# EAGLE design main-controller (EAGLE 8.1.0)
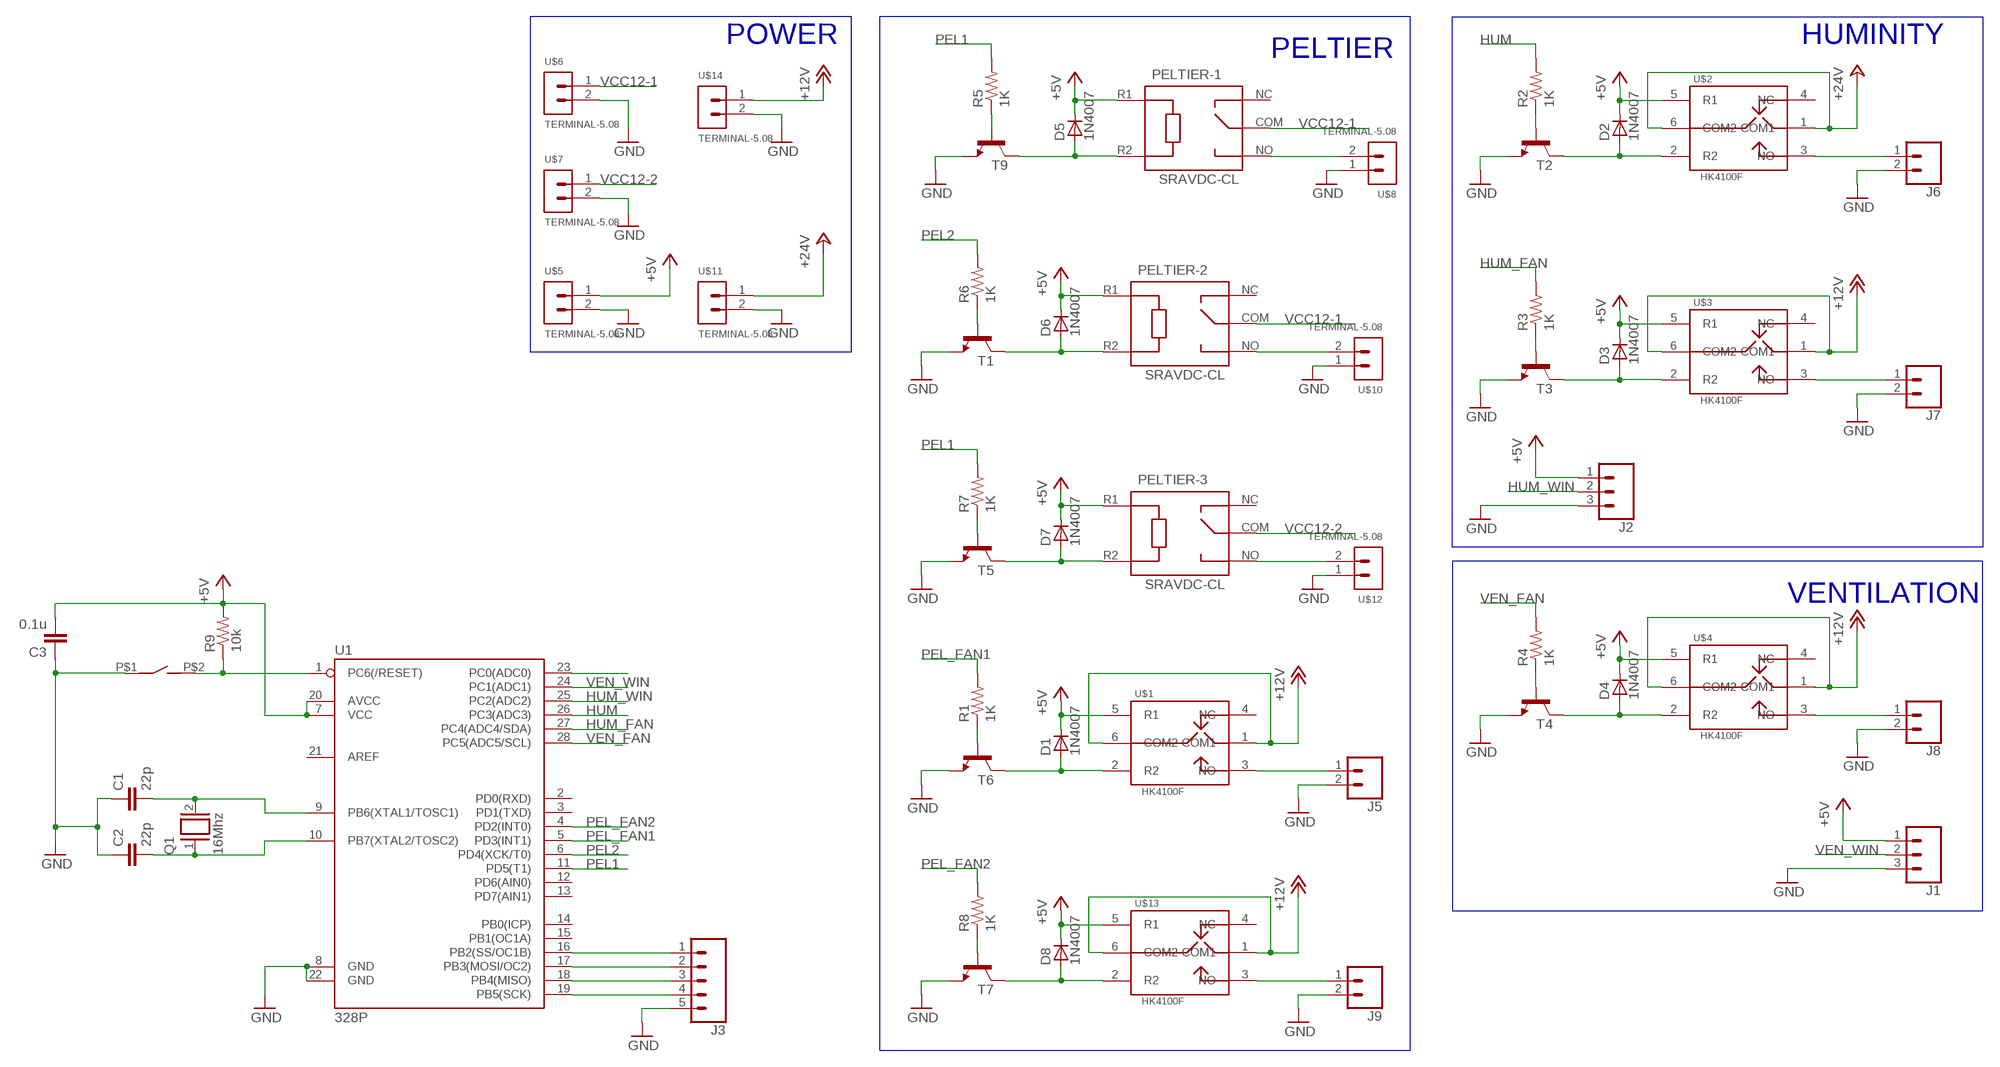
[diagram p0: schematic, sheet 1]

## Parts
C1  22p  C-EUC0805  [C0805]
C2  22p  C-EUC0805  [C0805]
C3  0.1u  C-EUC0805  [C0805]
D1  1N4007  [SMA]
D2  1N4007  [SMA]
D3  1N4007  [SMA]
D4  1N4007  [SMA]
D5  1N4007  [SMA]
D6  1N4007  [SMA]
D7  1N4007  [SMA]
D8  1N4007  [SMA]
J1  CONN_03  [1X03]
J2  CONN_03  [1X03]
J3  CONN_05KH2510  [1X05KF2510]
J5  CONN_02POLAR  [MOLEX-1X2]
J6  CONN_02POLAR  [MOLEX-1X2]
J7  CONN_02POLAR  [MOLEX-1X2]
J8  CONN_02POLAR  [MOLEX-1X2]
J9  CONN_02POLAR  [MOLEX-1X2]
PELTIER-1  SRAVDC-CL  [SRA-*VDC-CL]
PELTIER-2  SRAVDC-CL  [SRA-*VDC-CL]
PELTIER-3  SRAVDC-CL  [SRA-*VDC-CL]
Q1  16Mhz  XTAL/S  [QS]
R1  1K  R-US_M0805  [M0805]
R2  1K  R-US_M0805  [M0805]
R3  1K  R-US_M0805  [M0805]
R4  1K  R-US_M0805  [M0805]
R5  1K  R-US_M0805  [M0805]
R6  1K  R-US_M0805  [M0805]
R7  1K  R-US_M0805  [M0805]
R8  1K  R-US_M0805  [M0805]
R9  10k  R-US_R0805  [R0805]
T1  -NPN-SOT23-EBC  [SOT23-EBC]
T2  -NPN-SOT23-EBC  [SOT23-EBC]
T3  -NPN-SOT23-EBC  [SOT23-EBC]
T4  -NPN-SOT23-EBC  [SOT23-EBC]
T5  -NPN-SOT23-EBC  [SOT23-EBC]
T6  -NPN-SOT23-EBC  [SOT23-EBC]
T7  -NPN-SOT23-EBC  [SOT23-EBC]
T9  -NPN-SOT23-EBC  [SOT23-EBC]
U1  328P  ATMEGA328P_PDIP  [DIP28]
U$1  HK4100F  [HK4100F-DC5V-SHG]
U$2  HK4100F  [HK4100F-DC5V-SHG]
U$3  HK4100F  [HK4100F-DC5V-SHG]
U$4  HK4100F  [HK4100F-DC5V-SHG]
U$5  TERMINAL-5.08  [TERMINAL-5.08]
U$6  TERMINAL-5.08  [TERMINAL-5.08]
U$7  TERMINAL-5.08  [TERMINAL-5.08]
U$8  TERMINAL-5.08  [TERMINAL-5.08]
U$9  BUTTON  [BUTTON-2]
U$10  TERMINAL-5.08  [TERMINAL-5.08]
U$11  TERMINAL-5.08  [TERMINAL-5.08]
U$12  TERMINAL-5.08  [TERMINAL-5.08]
U$13  HK4100F  [HK4100F-DC5V-SHG]
U$14  TERMINAL-5.08  [TERMINAL-5.08]

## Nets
+5V: C3.2 D1.K(C) D2.K(C) D3.K(C) D4.K(C) D5.K(C) D6.K(C) D7.K(C) D8.K(C) J1.1 J2.1 PELTIER-1.R1 PELTIER-2.R1 PELTIER-3.R1 R9.2 U1.7(VCC) U1.20(AVCC) U$1.5(R1) U$2.5(R1) U$3.5(R1) U$4.5(R1) U$5.1 U$13.5(R1)
+12V: U$1.1(COM1) U$1.6(COM2) U$3.1(COM1) U$3.6(COM2) U$4.1(COM1) U$4.6(COM2) U$13.1(COM1) U$13.6(COM2) U$14.1
+24V: U$2.1(COM1) U$2.6(COM2) U$11.1
GND: C1.1 C2.1 C3.1 J1.3 J2.3 J3.5 J5.2 J6.2 J7.2 J8.2 J9.2 T1.E T2.E T3.E T4.E T5.E T6.E T7.E T9.E U1.8(GND) U1.22(GND) U$5.2 U$6.2 U$7.2 U$8.1 U$9.P$1 U$10.1 U$11.2 U$12.1 U$14.2
HUM: R2.2 U1.26(PC3(ADC3))
HUM_FAN: R3.2 U1.27(PC4(ADC4/SDA))
HUM_WIN: J2.2 U1.25(PC2(ADC2))
N$1: D1.A T6.C U$1.2(R2)
N$2: R6.1 T1.B
N$3: R2.1 T2.B
N$4: J5.1 U$1.3(NO)
N$5: D2.A T2.C U$2.2(R2)
N$6: R3.1 T3.B
N$7: R4.1 T4.B
N$8: J6.1 U$2.3(NO)
N$9: D3.A T3.C U$3.2(R2)
N$10: R1.1 T6.B
N$11: R7.1 T5.B
N$12: J7.1 U$3.3(NO)
N$13: D4.A T4.C U$4.2(R2)
N$14: R8.1 T7.B
N$15: C1.2 Q1.2 U1.9(PB6(XTAL1/TOSC1))
N$16: J8.1 U$4.3(NO)
N$17: D5.A PELTIER-1.R2 T9.C
N$18: R5.1 T9.B
N$19: C2.2 Q1.1 U1.10(PB7(XTAL2/TOSC2))
N$20: PELTIER-1.NO U$8.2
N$21: D6.A PELTIER-2.R2 T1.C
N$22: R9.1 U1.1(PC6(/RESET)) U$9.P$2
N$23: U1.23(PC0(ADC0))
N$24: PELTIER-2.NO U$10.2
N$25: D7.A PELTIER-3.R2 T5.C
N$27: J3.1 U1.16(PB2(SS/OC1B))
N$28: PELTIER-3.NO U$12.2
N$29: D8.A T7.C U$13.2(R2)
N$30: J3.2 U1.17(PB3(MOSI/OC2))
N$31: J3.3 U1.18(PB4(MISO))
N$32: J9.1 U$13.3(NO)
N$33: J3.4 U1.19(PB5(SCK))
PEL1: R5.2 R7.2 U1.11(PD5(T1))
PEL2: R6.2 U1.6(PD4(XCK/T0))
PEL_FAN1: R1.2 U1.5(PD3(INT1))
PEL_FAN2: R8.2 U1.4(PD2(INT0))
VCC12-1: PELTIER-1.COM PELTIER-2.COM U$6.1
VCC12-2: PELTIER-3.COM U$7.1
VEN_FAN: R4.2 U1.28(PC5(ADC5/SCL))
VEN_WIN: J1.2 U1.24(PC1(ADC1))
Unconnected: PELTIER-1.NC PELTIER-2.NC PELTIER-3.NC U1.2(PD0(RXD)) U1.3(PD1(TXD)) U1.12(PD6(AIN0)) U1.13(PD7(AIN1)) U1.14(PB0(ICP)) U1.15(PB1(OC1A)) U1.21(AREF) U$1.4(NC) U$2.4(NC) U$3.4(NC) U$4.4(NC) U$13.4(NC)

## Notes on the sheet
- POWER | HUMINITY
- PELTIER
- VENTILATION

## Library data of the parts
C1-C3 = resistor:C-EU: CAPACITOR, European symbol
D1-D8 = casovac:1N4007
J1 J2 = SparkFun-Connectors:CONN_03: Multi connection point. Often used as Generic Header-pin footprint for 0.1 inch spaced/style header connections On any of the 0.1 inch spaced packages, you can populate with these: Break Away Headers - Straight (PRT-00116) Break Away Male Headers - Right Angle (PRT-00553) Female Headers (PRT-00115)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
J3 = bon-connecters:CONN_05: Multi connection point. Often used as Generic Header-pin footprint for 0.1 inch spaced/style header connections On any of the 0.1 inch spaced packages, you can populate with these: Break Away Headers - Straight (PRT-00116) Break Away Male Headers - Right Angle (PRT-00553) Female Headers (PRT-00115)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
J5-J9 = SparkFun-Connectors:CONN_02: Multi connection point. Often used as Generic Header-pin footprint for 0.1 inch spaced/style header connections; SF_ID: PRT-09918
PELTIER-1-PELTIER-3 = huike:SRA*VDC-CL
Q1 = special:XTAL/S: CRYSTAL
R1-R9 = adafruit:R-US_: RESISTOR, American symbol
T1-T7 T9 = transistor:*-NPN-: NPN Transistror BF959 corrected 2008.03.06
U1 = SparkFun-IC-Microcontroller:ATMEGA328P_PDIP: Atmel 328P Through hole ATMEGA328P uC used in the Arduino 32kb flash, 1k EEPROM, 2k SRAM Datasheet SparkFun Products Storefront component: AVR 28 Pin 20MHz 32K 6A/D - ATMega328P (COM-09061) SparkFun Simon Says - Through-Hole Soldering Kit (KIT-10547) SparkFun Learn to Solder - Simon Says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; PROD_ID: IC-09136
U$1-U$4 U$13 = huike:HK4100F
U$5-U$8 U$10-U$12 U$14 = huike:TERMINAL-5.08
U$9 = huike:BUTTON

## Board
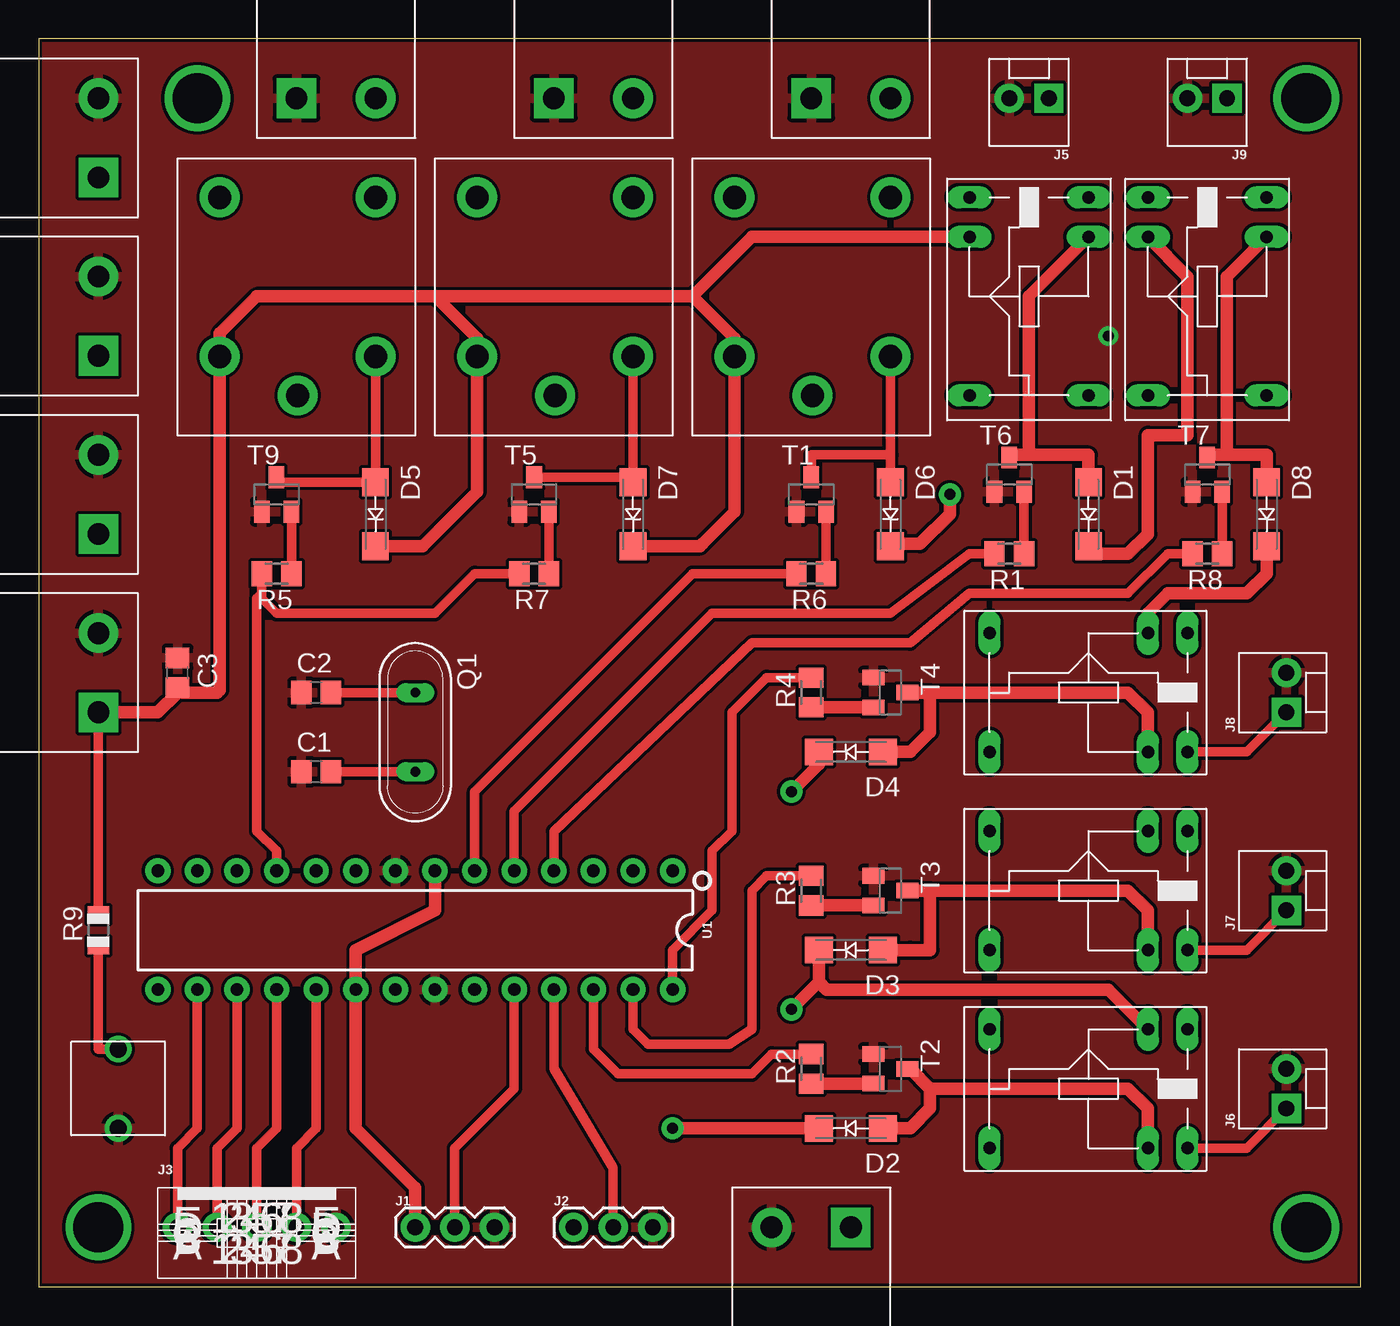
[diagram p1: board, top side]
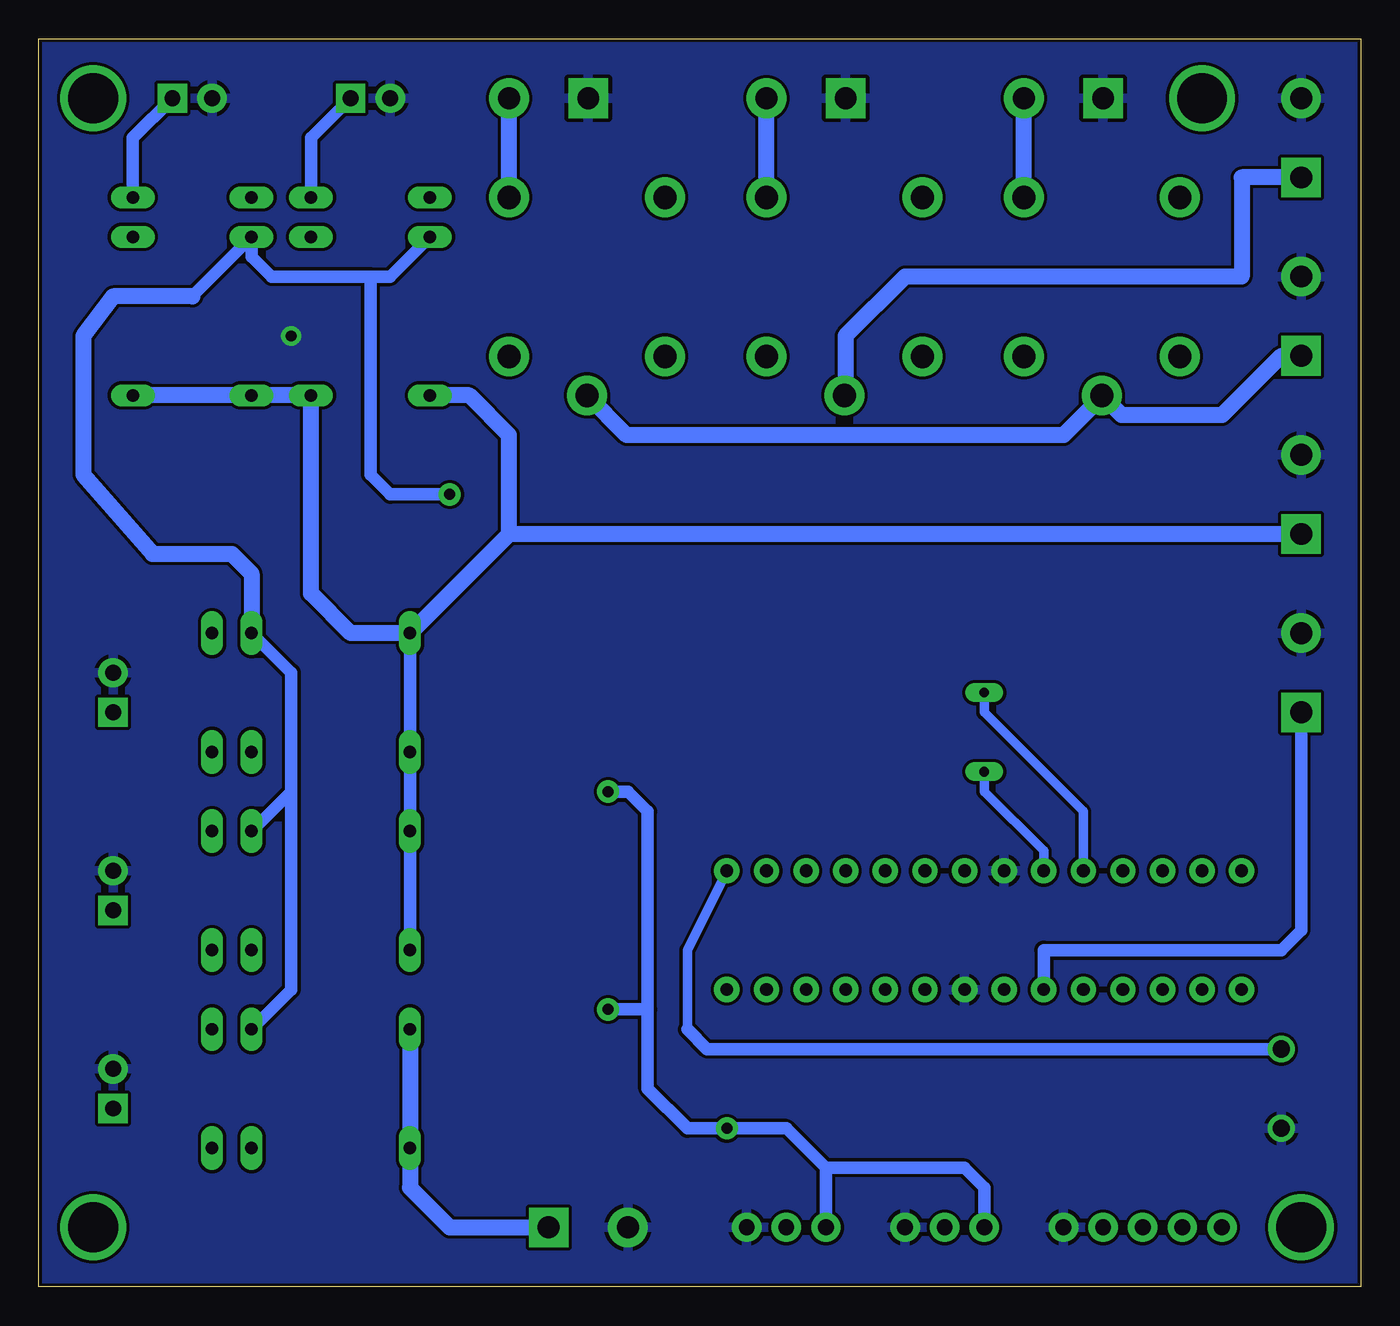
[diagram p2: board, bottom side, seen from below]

Size 84.76 x 80 mm. Coordinates in mm from the lower left corner, seen from the top.
Outline: 0,0 84.76,0 84.76,80 0,80 0,0
Copper layers (1*16): Top 0.035mm / dielectric 1.5mm / Bottom 0.035mm
Design rules "SparkFun *": minimum track width 8mil, minimum drill 20mil, track to track 8mil, track to pad 8mil, pad to pad 8mil, via to via 8mil, smd to smd 8mil, copper to edge 8mil, drill to drill 8mil, minimum pad ring 12mil, minimum via ring 10mil, stop-mask expansion 4mil, vias tented up to drill 20mil, thermal gap 10mil

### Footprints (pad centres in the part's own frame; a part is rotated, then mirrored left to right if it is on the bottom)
C0805 = smd 1.3 x 1.5: 1 -0.95,0; 2 0.95,0
SMA = smd 1.8 x 1.7: A -2.05,0; K 2.05,0
1X03 = drill 1.016 pad 1.88: 1 0,0; 2 2.54,0; 3 5.08,0
1X05KF2510 = drill 1.016 pad 1.88: 1 0,0; 2 2.54,0; 3 5.08,0; 4 7.62,0; 5 10.16,0
MOLEX-1X2 = drill 1.016 pad 1.88 square: 1 0,0 | drill 1.016 pad 1.88: 2 2.54,0
SRA-*VDC-CL = drill 1.5 pad 2.54: COM -2.5,5; NC 10.2,10; NO 10.2,0; R1 0,10; R2 0,0
QS = drill 0.61 long: 1 -2.54,0; 2 2.54,0
M0805 = smd 1.3 x 1.6: 1 -0.95,0; 2 0.95,0
R0805 = smd 1.1 x 1.4: 1 -1,0; 2 1,0
SOT23-EBC = smd 1 x 1.4: B 0.95,-1.1; C 0,1.1; E -0.95,-1.1
DIP28 = drill 0.813 pad 1.626: 1 -16.51,-3.81; 2 -13.97,-3.81; 3 -11.43,-3.81; 4 -8.89,-3.81; 5 -6.35,-3.81; 6 -3.81,-3.81; 7 -1.27,-3.81; 8 1.27,-3.81; 9 3.81,-3.81; 10 6.35,-3.81; 11 8.89,-3.81; 12 11.43,-3.81; 13 13.97,-3.81; 14 16.51,-3.81; 15 16.51,3.81; 16 13.97,3.81; 17 11.43,3.81; 18 8.89,3.81; 19 6.35,3.81; 20 3.81,3.81; 21 1.27,3.81; 22 -1.27,3.81; 23 -3.81,3.81; 24 -6.35,3.81; 25 -8.89,3.81; 26 -11.43,3.81; 27 -13.97,3.81; 28 -16.51,3.81
HK4100F-DC5V-SHG = drill 0.8 pad 1.27 long: 1 1.27,1.27; 2 11.43,1.27; 3 13.97,1.27; 4 13.97,8.89; 5 11.43,8.89; 6 1.27,8.89
TERMINAL-5.08 = drill 1.4 pad 2.54 square: 1 0,0 | drill 1.4 pad 2.54: 2 5.08,0
BUTTON-2 = drill 1.1 pad 1.676: P$1 0,0; P$2 5.08,0

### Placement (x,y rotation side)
C1  17.78,33.02 0 top
C2  17.78,38.1 0 top
C3  8.89,39.37 270 top
D1  67.31,49.53 270 top
D2  52.07,10.16 180 top
D3  52.07,21.59 180 top
D4  52.07,34.29 180 top
D5  21.59,49.53 270 top
D6  54.61,49.53 270 top
D7  38.1,49.53 270 top
D8  78.74,49.53 270 top
J1  24.13,3.81 0 top
J2  34.29,3.81 0 top
J3  8.89,3.81 0 top
J5  64.77,76.2 180 top
J6  80.01,11.43 90 top
J7  80.01,24.13 90 top
J8  80.01,36.83 90 top
J9  76.2,76.2 180 top
PELTIER-1  21.59,59.65 90 top
PELTIER-2  54.61,59.65 90 top
PELTIER-3  38.1,59.65 90 top
Q1  24.13,35.56 270 top
R1  62.23,46.99 180 top
R2  49.53,13.97 90 top
R3  49.53,25.4 90 top
R4  49.53,38.1 90 top
R5  15.24,45.72 180 top
R6  49.53,45.72 180 top
R7  31.75,45.72 180 top
R8  74.93,46.99 180 top
R9  3.81,22.86 90 top
T1  49.53,50.8 0 top
T2  54.61,13.97 270 top
T3  54.61,25.4 270 top
T4  54.61,38.1 270 top
T5  31.75,50.8 0 top
T6  62.23,52.07 0 top
T7  74.93,52.07 0 top
T9  15.24,50.8 0 top
U1  24.13,22.86 180 top
U$1  68.58,55.88 90 top
U$2  59.69,7.62 0 top
U$3  59.69,20.32 0 top
U$4  59.69,33.02 0 top
U$5  3.81,36.83 90 top
U$6  3.81,59.69 90 top
U$7  3.81,71.12 90 top
U$8  16.51,76.2 0 top
U$9  5.08,10.16 90 top
U$10  49.53,76.2 0 top
U$11  52.07,3.81 180 top
U$12  33.02,76.2 0 top
U$13  80.01,55.88 90 top
U$14  3.81,48.26 90 top

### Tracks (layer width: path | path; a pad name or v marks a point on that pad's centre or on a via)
+5V  (via drill 0.7 pad 1.42)
  Top 0.61: U$5.1 R9.2
  Top 0.813: 25.4,63.5 13.97,63.5 11.59,61.12 PELTIER-1.R1 11.59,38.26 11.43,38.1 9.21,38.1 C3.2 8.89,38.1 7.62,36.83 U$5.1 | D5.K 24.62,47.48 28.1,50.96 PELTIER-3.R1 28.1,60.8 25.4,63.5 | U$4.5 71.12,43.18 72.39,44.45 77.47,44.45 78.74,45.72 D8.K | 41.91,63.5 45.72,67.31 U$1.5 | 25.4,63.5 41.91,63.5 | 38.59,46.99 D7.K 42.4,47.48 42.55,47.62 44.61,49.69 PELTIER-2.R1 44.61,60.8 41.91,63.5 | D1.K 67.8,46.99 69.85,46.99 71.12,48.26 71.12,54.61 73.66,54.61 73.66,64.77 U$13.5 | D3.K 50.02,19.54 | v48.26,31.75 50.02,33.51 D4.K | U$2.5 68.58,19.05 50.51,19.05 50.02,19.54 | v58.42,50.8 58.42,49.53 56.52,47.62 54.76,47.62 D6.K | U1.7 25.4,24.13 20.32,21.59 U1.20 20.32,10.16 24.13,6.35 J1.1 | v40.64,10.16 D2.K | 50.02,19.54 v48.26,17.78
  Bottom 0.813: U$4.5 68.58,39.37 68.58,31.75 | 68.58,31.75 U$3.5 | U$1.5 62.23,64.77 63.5,64.77 | 63.5,64.77 69.85,64.77 71.12,66.04 U$13.5 74.93,63.5 | 68.58,31.75 68.58,19.05 U$2.5 | v48.26,31.75 46.99,31.75 45.72,30.48 45.72,17.78 | v58.42,50.8 62.23,50.8 63.5,52.07 63.5,64.77 | U1.20 20.32,21.59 5.08,21.59 3.81,22.86 U$5.1 | J2.1 34.29,7.62 | J1.1 24.13,6.35 25.4,7.62 34.29,7.62 | 45.72,17.78 45.72,12.7 43.18,10.16 v40.64,10.16 36.83,10.16 34.29,7.62 | v48.26,17.78 45.72,17.78
  Bottom 1.016: 74.93,63.5 80.01,63.5 81.92,60.96 81.92,52.07 77.47,46.99 72.39,46.99 71.12,45.72 U$4.5
+12V
  Bottom 0.813: U$3.1 U$3.6 U$4.1 U$4.6
  Bottom 1.016: U$14.1 50.8,48.26 54.61,48.26 | 54.61,48.26 U$4.6 64.77,41.91 67.31,44.45 U$1.1 U$13.6 U$13.1 | 54.61,48.26 54.61,54.61 57.15,57.15 U$1.6
+24V
  Bottom 1.016: U$11.1 58.42,3.81 60.96,6.35 U$2.1 U$2.6
GND  (via drill 0.7 pad 1.27)
  other vias: 68.58,60.96
  pour Bottom: 0,0 0,80.01 85.09,80.01 85.09,0
  pour Top: 0,0 0,80.01 85.09,80.01 85.09,0
HUM
  Top 0.61: U1.26 35.56,15.24 37.15,13.65 45.72,13.65 46.99,14.92 R2.2
HUM_FAN
  Top 0.61: R3.2 46.67,26.35 45.72,25.4 45.72,16.51 44.26,15.53 39.08,15.53 38.1,16.51 U1.27
HUM_WIN
  Top 0.61: J2.2 36.83,7.62 33.02,13.97 U1.25
N$1
  Top 0.813: D1.A 67.31,53.34 63.5,53.34 | 63.5,53.34 62.4,53.34 T6.C | 63.5,53.34 63.5,63.5 U$1.2
N$2
  Top 0.61: T1.B R6.1
N$3
  Top 0.813: R2.1 T2.B
N$4
  Bottom 0.813: U$1.3 67.31,73.66 J5.1
N$5
  Top 0.813: 57.15,12.7 69.85,12.7 71.12,11.43 U$2.2 | 57.15,12.7 55.88,13.97 T2.C | 57.15,12.7 57.15,11.43 55.88,10.16 D2.A
N$6
  Top 0.813: R3.1 T3.B
N$7
  Top 0.813: R4.1 T4.B
N$8
  Top 0.61: U$2.3 77.47,8.89 J6.1
N$9
  Top 0.813: 55.88,21.59 D3.A 55.88,21.59 | T3.C 57.15,25.4 | 55.88,21.59 57.15,21.59 57.15,25.4 | 57.15,25.4 69.85,25.4 71.12,24.13 U$3.2
N$10
  Top 0.61: T6.B R1.1
N$11
  Top 0.61: R7.1 T5.B
N$12
  Top 0.61: U$3.3 77.47,21.59 J7.1
N$13
  Top 0.813: 57.15,38.1 T4.C | 57.15,38.1 69.85,38.1 71.12,36.83 U$4.2 | D4.A 55.88,34.29 57.15,35.56 57.15,38.1
N$14
  Top 0.61: T7.B R8.1
N$15
  Top 0.61: C1.2 Q1.2
  Bottom 0.61: U1.9 20.32,27.94 24.13,31.75 Q1.2
N$16
  Top 0.61: U$4.3 77.47,34.29 J8.1
N$17
  Top 0.61: PELTIER-1.R2 D5.A 15.24,51.58 T9.C
N$18
  Top 0.61: R5.1 T9.B
N$19
  Top 0.61: C2.2 Q1.1
  Bottom 0.61: U1.10 17.78,30.48 24.13,36.83 Q1.1
N$20
  Bottom 1.016: PELTIER-1.NO U$8.2
N$21
  Top 0.61: D6.A 54.61,53.34 | 54.61,53.34 49.53,53.34 T1.C | 54.61,53.34 PELTIER-2.R2
N$22
  Top 0.61: R9.1 3.81,15.24 U$9.P$2
  Bottom 0.61: U1.1 43.18,21.59 43.18,16.51
  Bottom 0.813: 43.18,16.51 41.91,15.24 U$9.P$2
N$24
  Bottom 1.016: PELTIER-2.NO U$10.2
N$25
  Top 0.61: 38.1,52.07 PELTIER-3.R2 | D7.A 38.1,51.9 38.1,52.07 | T5.C 37.93,51.9 38.1,52.07
N$26  (via drill 3.2 pad 3.81)
  other vias: 81.28,76.2
N$27
  Top 0.61: J3.1 8.89,8.89 10.16,10.16 U1.16
N$28
  Bottom 1.016: PELTIER-3.NO U$12.2
N$29
  Top 0.813: D8.A 78.74,53.34 76.2,53.34 | 76.2,53.34 75.1,53.34 T7.C | 76.2,53.34 76.2,64.77 U$13.2
N$30
  Top 0.61: J3.2 11.43,8.89 12.7,10.16 U1.17
N$31
  Top 0.61: J3.3 13.97,8.89 15.24,10.16 U1.18
N$32
  Bottom 0.813: U$13.3 78.74,73.66 J9.1
N$33
  Top 0.61: J3.4 16.51,8.89 17.78,10.16 U1.19
N$34  (via drill 3.2 pad 3.81)
  other vias: 10.16,76.2
N$35  (via drill 3.2 pad 3.81)
  other vias: 81.28,3.81
N$36  (via drill 3.2 pad 3.81)
  other vias: 3.81,3.81
PEL1
  Top 0.61: R7.2 27.94,45.72 25.4,43.18 15.24,43.18 14.29,44.13 14.29,44.45 | R5.2 14.29,44.45 | 14.29,44.45 13.97,44.13 13.97,29.21 15.24,27.94 U1.11
PEL2
  Top 0.61: R6.2 41.91,45.72 27.94,31.75 U1.6
PEL_FAN1
  Top 0.61: U1.5 30.48,30.48 43.18,43.18 54.61,43.18 59.69,46.99 R1.2
PEL_FAN2
  Top 0.61: R8.2 72.39,46.99 69.85,44.45 59.69,44.45 55.88,41.27 45.72,41.27 33.02,29.21 U1.4
VCC12-1
  Bottom 1.016: U$6.1 5.08,59.69 8.89,55.88 15.32,55.88 PELTIER-1.COM 16.59,57.07 19.05,54.61 47.07,54.61 PELTIER-2.COM
VCC12-2
  Bottom 1.016: U$7.1 7.62,71.12 7.62,64.77 29.21,64.77 33.02,60.96 33.02,57.23 PELTIER-3.COM
VEN_FAN
  Top 0.61: R4.2 46.67,39.05 44.45,36.83 44.45,29.21 43.18,27.94 43.18,24.13 40.64,21.59 U1.28
VEN_WIN
  Top 0.61: U1.24 30.48,12.7 26.67,8.89 J1.2

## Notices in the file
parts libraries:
SparkFun-Connectors: Licensing: Creative Commons ShareAlike 4.0 International - https://creativecommons.org/licenses/by-sa/4.0
